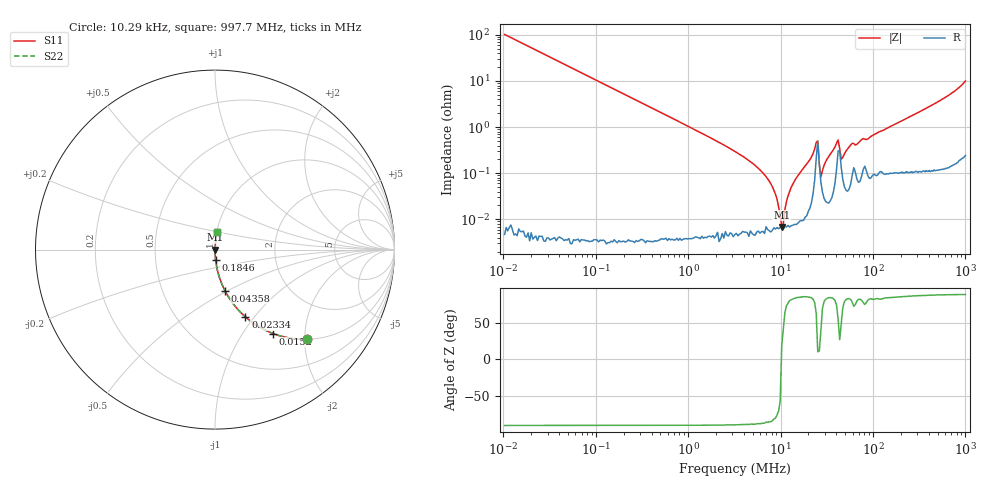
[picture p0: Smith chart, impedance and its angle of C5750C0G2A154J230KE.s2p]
! S-Parameter Data Generated by TDK Corporation
! Copyright(C) 2025 TDK Corporation.
! All Rights Reserved.
! TDK P/N: C5750C0G2A154J230KE (Multilayer Ceramic Chip Capacitor)
! Property: C=150nF
! Size(LxWxT): 5.7x5x2.3mm
! Model Type: s2p (Touchstone File Format Version 1.0)
! Frequency: DC=Yes Start=0.01028704MHz Stop=997.7393MHz 352points Log-sweep
! Model Generated on July 30, 2025
! Terms and conditions regarding TDK Simulation Models:
! 1)This simulation model is being provided solely for informational
!  purposes. Please refer to the specifications of the products in
!  terms of detailed characteristics of such products.
! 2)In no event shall TDK Corporation of any of its subsidiaries be
!  liable for any loss or damage arising, directly or indirectly,
!  from any information contained in this simulation model, including,
!  but not limited to loss or damages arising from any inaccuracies,
!  omissions or errors in connection with such information.
! 3)Any and all copyrights on this simulation model are owned by
!  TDK Corporation.  Duplication or redistribution of this simulation
!  model without prior written permission from TDK Corporation
!  is prohibited.
! 4)This simulation model is subject to any modification or change
!  without any prior notice.
! 5)Neither TDK Corporation nor any of its subsidiaries shall make any
!  warranty, express or implied, including but not limited to the
!  correctness, implied warranties of merchantability and fitness for
!  a particular purpose with respect to this simulation models.
! 6)The use of this simulation model shall be deemed to have consented
!  to the terms and conditions hereof.
! Port Assignments:
!  1 ---| |--- 2
! Applicable Conditions:
!  Temperature = 25 degC
!  DC Bias Voltage = 0 V
!  Small Signal Operation
# Hz S MA R 50
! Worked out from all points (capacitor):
!   351 points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, 10.29 kHz to 997.7 MHz, reference 50 ohm
!   read as one part in series: C = 151 nF near 10.7 kHz
!   lowest |Z| = 6.85 mohm at 10.27 MHz (marker M1)
!   series resonance near 10.2 MHz, so ESL is about 1.6 nH
!   S11 on the Smith chart (normalised r, x): 10.29 kHz: 1.00, -2.05; 15.2 kHz: 1.00, -1.39; 23.34 kHz: 1.00, -0.90; 43.58 kHz: 1.00, -0.48; 184.6 kHz: 1.00, -0.11; 997.7 MHz: 1.00, +0.20
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10287.04  0.7153 -44.3  0.6988 45.7  0.6988 45.7  0.7153 -44.3
15196.53  0.5695 -55.3  0.8219 34.7  0.8219 34.7  0.5695 -55.3
23342.29  0.4112 -65.7  0.9115 24.3  0.9115 24.3  0.4112 -65.7
43578.22  0.2349 -76.4  0.972 13.6  0.972 13.6  0.2349 -76.4
72370.14  0.144 -81.7  0.9895 8.3  0.9895 8.3  0.144 -81.7
184607.1  0.05692 -86.7  0.9983 3.3  0.9983 3.3  0.05692 -86.7
489646.8  0.02145 -88.7  0.9997 1.2  0.9997 1.2  0.02145 -88.7
3312886  0.002849 -88.8  0.9999 0.2  0.9999 0.2  0.002849 -88.8
7229596  0.0007558 -85.4  0.9999 0.0  0.9999 0.0  0.0007558 -85.4
8787006  0.0003509 -79.9  0.9999 0.0  0.9999 0.0  0.0003509 -79.9
1.027123e7  6.848e-05 19.0  0.9999 -0.0  0.9999 -0.0  6.848e-05 19.0
1.067992e7  8.19e-05 41.7  0.9999 -0.0  0.9999 -0.0  8.19e-05 41.7
1.29806e7  0.0004939 81.5  0.9999 -0.0  0.9999 -0.0  0.0004939 81.5
2.241455e7  0.002668 82.0  0.9996 -0.2  0.9996 -0.2  0.002668 82.0
2.5198e7  0.004996 10.4  0.9951 -0.1  0.9951 -0.1  0.004996 10.4
2.724312e7  0.0008304 39.3  0.9994 -0.0  0.9994 -0.0  0.0008304 39.3
3.062619e7  0.001779 82.0  0.9998 -0.1  0.9998 -0.1  0.001779 82.0
4.18462e7  0.005247 54.4  0.997 -0.2  0.997 -0.2  0.005247 54.4
4.524252e7  0.00201 48.5  0.9987 -0.1  0.9987 -0.1  0.00201 48.5
5.945172e7  0.004451 78.1  0.9991 -0.2  0.9991 -0.2  0.004451 78.1
1.49005e8  0.009993 83.8  0.999 -0.6  0.999 -0.6  0.009993 83.8
9.977393e8  0.09983 82.9  0.9926 -5.7  0.9926 -5.7  0.09983 82.9
